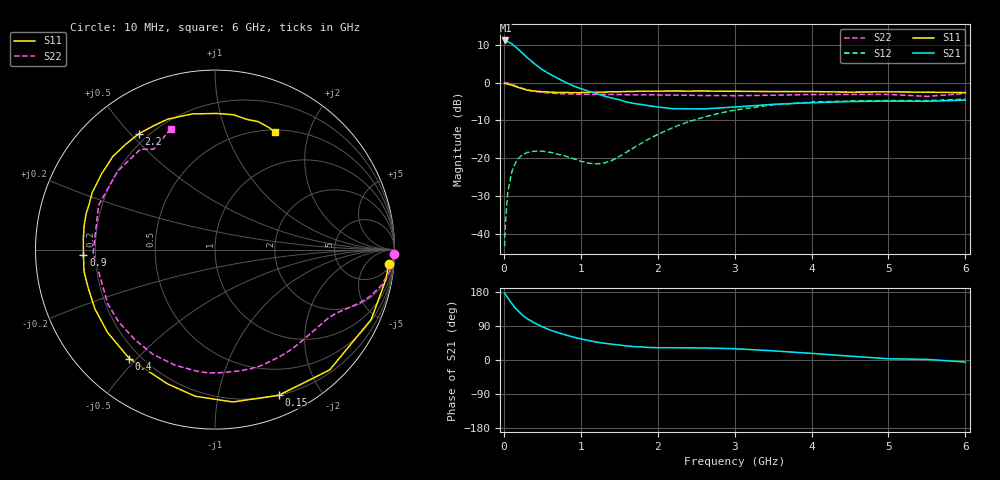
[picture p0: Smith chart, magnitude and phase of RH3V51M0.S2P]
! SIEMENS Small Signal Semiconductors
! BFR106
! Si NPN RF Bipolar Junction Transistor in SOT23
! VCE = 3.5 V  IC = 1 mA
! Common Emitter S-Parameters:  August  1996
# GHz  S  MA  R  50
!  f  S11  S21  S12  S22
! GHz  MAG  ANG  MAG  ANG  MAG  ANG  MAG  ANG
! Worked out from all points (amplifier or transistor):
!   36 points, 10 MHz to 6 GHz, reference 50 ohm
!   highest |S21| = 11.1 dB at 20 MHz (marker M1)
!   |S21| within 3 dB of that: start of sweep to 222.5 MHz
!   unconditionally stable (mu >= 1): 860.6 MHz to 2.167 GHz; 2.354 GHz to end of sweep
!   at 250 MHz: K = 0.27, MSG = 13.3 dB, |S12| = -19.0 dB
!   at 1.4 GHz: K = 1.44, MAG = 4.3 dB, |S12| = -20.7 dB
!   at 6 GHz: K = 1.02, MAG = -1.0 dB, |S12| = -4.4 dB
!   S11 on the Smith chart (normalised r, x): 10 MHz: 8, -21; 150 MHz: 0.20, -1.51; 400 MHz: 0.16, -0.48; 900 MHz: 0.15, -0.02; 2.2 GHz: 0.16, +0.53; 6 GHz: 0.52, +1.50
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0.01  0.9701 -4.8  3.599 176.3  0.0068 89.4  0.9996 -1.4
0.02  0.9668 -9.9  3.607 173.9  0.0137 84.5  0.997 -2.6
0.05  0.9534 -24.1  3.482 163.9  0.0343 75.8  0.983 -6.4
0.1  0.9262 -46.4  3.27 150.2  0.0642 64.4  0.9508 -11.9
0.15  0.8856 -66.4  2.976 136.5  0.0863 53.0  0.9057 -16.5
0.2  0.8548 -83.3  2.68 126.6  0.1016 44.8  0.8673 -19.6
0.25  0.8246 -97.7  2.407 116.9  0.1121 37.7  0.8289 -22.3
0.3  0.7931 -109.6  2.157 109.6  0.1181 32.6  0.8012 -24.3
0.4  0.7723 -128.2  1.767 97.7  0.1237 24.6  0.7617 -27.8
0.5  0.7561 -142.3  1.479 87.5  0.1229 19.4  0.7384 -31.0
0.6  0.7461 -153.6  1.289 79.2  0.1194 16.2  0.7242 -34.6
0.9  0.7336 -177.5  0.907 60.7  0.0985 17.6  0.7028 -46.1
1.1  0.7412 169.8  0.769 51.5  0.0855 28.1  0.6988 -54.8
1.3  0.7459 159.5  0.665 44.4  0.0857 47.0  0.6945 -63.7
1.6  0.7601 146.2  0.551 37.0  0.1205 68.8  0.6899 -78.0
2.2  0.7726 123.3  0.45 32.3  0.2539 71.3  0.6813 -109.1
2.8  0.7668 104.5  0.46 30.9  0.3911 56.9  0.6712 -142.9
3.5  0.7586 89.5  0.514 24.2  0.5077 38.2  0.6789 -178.7
4.5  0.7467 76.1  0.56 10.1  0.5681 15.8  0.6966 141.1
5  0.7527 71.4  0.566 3.3  0.5758 7.6  0.6969 126.6
5.5  0.7436 66.2  0.564 1.6  0.5778 3.8  0.6548 121.4
6  0.736 63.2  0.585 -5.4  0.6008 -4.0  0.7165 110.2
